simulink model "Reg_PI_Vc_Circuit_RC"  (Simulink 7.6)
settings: Solver=ode15s  StartTime=0.0  StopTime=40  RelTol=1e-3
InitFcn:
  | clc, close all
  | Kp=1.02;
  | R1=10e3;
  | R2=(Kp-1)*R1;
  | 
  | Ti=0.01;
  | C2=Ti/(R1+R2);
  | 
  | % circuit R C
  | R=10e3;
  | C=1e-3;
StopFcn:
  | close all, clc
  | load reg_PI.mat
  | plot(x(1,:),x(2,:),x(1,:),x(3,:),x(1,:),x(4,:))
  | title('Signaux de consigne, commande et sortie')
  | xlabel('temps')
  | grid
libraries: fl_lib x12, nesl_utility x4, elec_lib x1

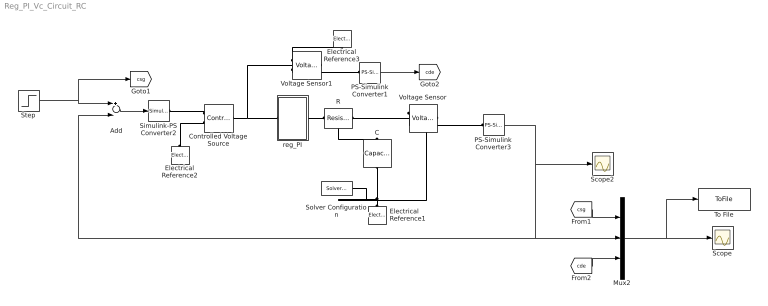
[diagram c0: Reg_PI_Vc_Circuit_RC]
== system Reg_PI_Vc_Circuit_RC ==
  Add : Sum  Inputs=+-
  C : fl_lib/Electrical/Electrical Elements/Capacitor  DialogController=NetworkEngine.DynNeDlgSource  SystemSampleTime=-1  c=C F  v0=0 V  r=1e-22 Ohm  g=0 1/Ohm  i_Log=off  v_Log=off  vc_Log=off  LocalVarNames=|i|v|vc  LocalVarDescs=|i|v|Internal variable for voltage across capacitor term  LocalVarLogging=[0 0 0]
  Controlled Voltage Source : fl_lib/Electrical/Electrical Sources/Controlled Voltage Source  DialogController=NetworkEngine.DynNeDlgSource  SystemSampleTime=-1  i_Log=off  v_Log=off  LocalVarNames=|i|v  LocalVarDescs=|i|v  LocalVarLogging=[0 0]
  Electrical Reference1 : fl_lib/Electrical/Electrical Elements/Electrical Reference  DialogController=NetworkEngine.DynNeDlgSource  SystemSampleTime=-1  i_Log=off  LocalVarNames=|i  LocalVarDescs=|i  LocalVarLogging=[]
  Electrical Reference2 : fl_lib/Electrical/Electrical Elements/Electrical Reference  DialogController=NetworkEngine.DynNeDlgSource  SystemSampleTime=-1  i_Log=off  LocalVarNames=|i  LocalVarDescs=|i  LocalVarLogging=[]
  Electrical Reference3 : fl_lib/Electrical/Electrical Elements/Electrical Reference  DialogController=NetworkEngine.DynNeDlgSource  SystemSampleTime=-1  i_Log=off  LocalVarNames=|i  LocalVarDescs=|i  LocalVarLogging=[]
  Mux2 : Mux  Inputs=3
  PS-Simulink Converter1 : nesl_utility/PS-Simulink Converter  DialogController=NetworkEngine.DynNeUtilDlgSource  SystemSampleTime=-1  PhysicalDomain=network_engine_domain  LeftPortType=input  RightPortType=output  SubClassName=ps_output  Unit=V  AffineConversion=off
  PS-Simulink Converter3 : nesl_utility/PS-Simulink Converter  DialogController=NetworkEngine.DynNeUtilDlgSource  SystemSampleTime=-1  PhysicalDomain=network_engine_domain  LeftPortType=input  RightPortType=output  SubClassName=ps_output  Unit=V  AffineConversion=off
  R : fl_lib/Electrical/Electrical Elements/Resistor  DialogController=NetworkEngine.DynNeDlgSource  SystemSampleTime=-1  R=R Ohm  i_Log=off  v_Log=off  LocalVarNames=|i|v  LocalVarDescs=|i|v  LocalVarLogging=[0 0]
  Scope : Scope
  Scope2 : Scope
  Simulink-PS Converter2 : nesl_utility/Simulink-PS Converter  DialogController=NetworkEngine.DynNeUtilDlgSource  SystemSampleTime=-1  PhysicalDomain=network_engine_domain  LeftPortType=input  RightPortType=output  SubClassName=ps_input  Unit=1  AffineConversion=off  InputFilterTimeConstant=.001  UdotUserProvided=0
  Solver Configuration : nesl_utility/Solver Configuration  DialogController=NetworkEngine.DynNeUtilDlgSource  SystemSampleTime=-1  PhysicalDomain=network_engine_domain  LeftPortType=input  RightPortType=generic  SubClassName=solver  Accelerate=off  Profile=off  ResidualTolerance=1e-9  MaxNonlinIter=12  MaxModeIter=2  DoFixedCost=off  UseLocalSampling=off  DoDC=off  LinearAlgebra=Sparse  LocalSolverSampleTime=.001  LocalSolverChoice=NE_BACKWARD_EULER_ADVANCER  UseLocalSolver=off
  Step : Step  Time=5  After=5  SampleTime=0
  To File : ToFile  Filename=reg_PI  MatrixName=x
  Voltage Sensor : fl_lib/Electrical/Electrical Sensors/Voltage Sensor  DialogController=NetworkEngine.DynNeDlgSource  SystemSampleTime=-1  i1_Log=off  v1_Log=off  LocalVarNames=|i1|v1  LocalVarDescs=|i1|v1  LocalVarLogging=[0 0]
  Voltage Sensor1 : fl_lib/Electrical/Electrical Sensors/Voltage Sensor  DialogController=NetworkEngine.DynNeDlgSource  SystemSampleTime=-1  i1_Log=off  v1_Log=off  LocalVarNames=|i1|v1  LocalVarDescs=|i1|v1  LocalVarLogging=[0 0]
  reg_PI : Subsystem
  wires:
  Add/1 -> Simulink-PS Converter2/1
  Step/1 -> Add/1, [csg]
  PS-Simulink Converter3/1 -> Scope2/1, Add/2, Mux2/2
  Mux2/1 -> Scope/1, To File/1
  PS-Simulink Converter1/1 -> [cde]
  [cde] -> Mux2/3
  [csg] -> Mux2/1
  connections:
  Controlled Voltage Source/RConn1 -- Simulink-PS Converter2/RConn1
  Electrical Reference2/LConn1 -- Controlled Voltage Source/RConn2
  Controlled Voltage Source/LConn1 -- reg_PI/LConn1 -- Voltage Sensor1/LConn1
  reg_PI/RConn1 -- R/RConn1
  R/LConn1 -- C/LConn1 -- Voltage Sensor/LConn1
  Electrical Reference1/LConn1 -- C/RConn1 -- Voltage Sensor/RConn2 -- Solver Configuration/RConn1
  Voltage Sensor/RConn1 -- PS-Simulink Converter3/LConn1
  Voltage Sensor1/RConn1 -- PS-Simulink Converter1/LConn1
  Voltage Sensor1/RConn2 -- Electrical Reference3/LConn1

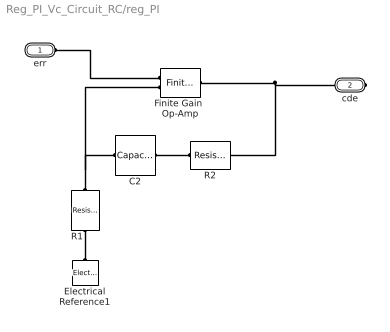
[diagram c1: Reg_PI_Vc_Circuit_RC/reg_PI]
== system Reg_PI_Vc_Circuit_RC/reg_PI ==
  C2 : fl_lib/Electrical/Electrical Elements/Capacitor  DialogController=NetworkEngine.DynNeDlgSource  SystemSampleTime=-1  c=C2 F  v0=0 V  r=1e-22 Ohm  g=0 1/Ohm  i_Log=off  v_Log=off  vc_Log=off  LocalVarNames=|i|v|vc  LocalVarDescs=|i|v|Internal variable for voltage across capacitor term  LocalVarLogging=[0 0 0]
  Electrical Reference1 : fl_lib/Electrical/Electrical Elements/Electrical Reference  DialogController=NetworkEngine.DynNeDlgSource  SystemSampleTime=-1  i_Log=off  LocalVarNames=|i  LocalVarDescs=|i  LocalVarLogging=[]
  Finite Gain  Op-Amp : elec_lib/Integrated Circuits/Finite Gain Op-Amp  DialogController=NetworkEngine.DynNeDlgSource  SystemSampleTime=-1  A=1000  Rin=1e+6 Ohm  Rout=100 Ohm  Vmin=-15 V  Vmax=15 V  LocalVarLogging=[]
  R1 : fl_lib/Electrical/Electrical Elements/Resistor  DialogController=NetworkEngine.DynNeDlgSource  SystemSampleTime=-1  R=R1 Ohm  i_Log=off  v_Log=off  LocalVarNames=|current|voltage|power  LocalVarDescs=|Resistor current (A)|Voltage across resistor (V)|Power (W)  LocalVarLogging=[0 0 0]
  R2 : fl_lib/Electrical/Electrical Elements/Resistor  DialogController=NetworkEngine.DynNeDlgSource  SystemSampleTime=-1  R=R2 Ohm  i_Log=off  v_Log=off  LocalVarNames=|current|voltage|power  LocalVarDescs=|Resistor current (A)|Voltage across resistor (V)|Power (W)  LocalVarLogging=[0 0 0]
  err : PMIOPort  Port=1  Side=Left
  cde : PMIOPort  Port=2  Side=Right
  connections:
  err/RConn1 -- Finite Gain  Op-Amp/LConn1
  R1/LConn1 -- Electrical Reference1/LConn1
  C2/RConn1 -- R2/LConn1
  R1/RConn1 -- Finite Gain  Op-Amp/LConn2 -- C2/LConn1
  Finite Gain  Op-Amp/RConn1 -- cde/RConn1 -- R2/RConn1
